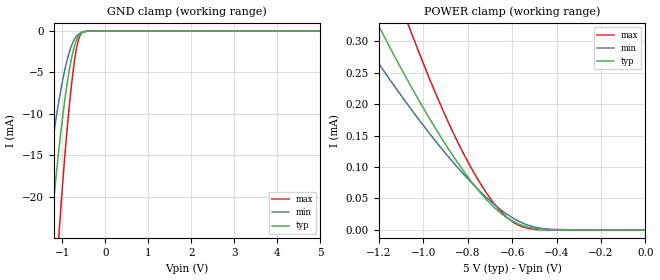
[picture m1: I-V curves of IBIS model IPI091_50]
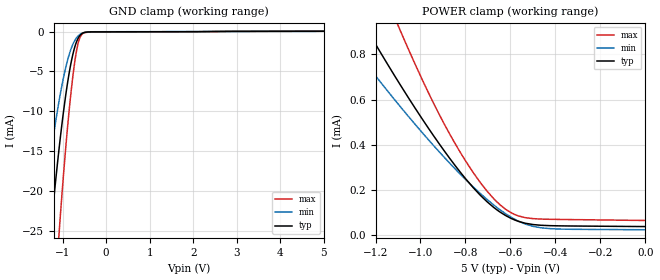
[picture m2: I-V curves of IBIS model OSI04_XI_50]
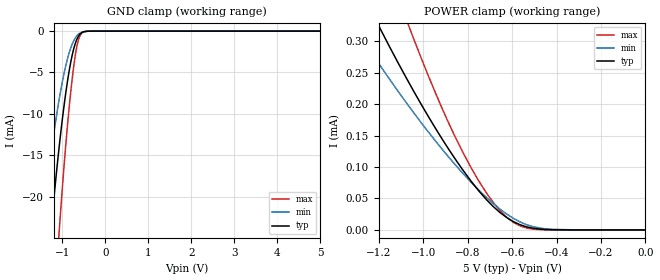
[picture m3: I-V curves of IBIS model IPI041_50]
| TEXAS INSTRUMENTS INCORPORATED
| Connectivity Solutions Group
| IBIS Model of TL16CP752CRHB_5V
| P752C_RHB_5V
| This file contains package information for the following:
|  QFP 32-pin (QFP) package as [Component] P752CRHB_5V
| This device can be powered at the following Vccs:
|  5 Volt Vcc
| This file provides unique models under the [Model Selector] for each Vcc.
| For operation at a specific Vcc, select the appropriate model after each
| [Model Selector] keyword.
[IBIS Ver]   3.2
[Comment char]  |_char
[File Name]   752c_rhb_5v.ibs
[File Rev]   1 | a
[Date]   December 5, 2007
[Source]   Data created from TI-SPICE simulations at TI-CONN.
[Notes]   The following is an IBIS list for the P754C_PM_5V.
   Please contact s-ly@ti.com with questions and
   comments concerning CONN IBIS models.
[Disclaimer] Property of Texas Instruments Incorporated.  Unauthorized
   reproduction and/or distribution is strictly prohibited.
   This product is protected under copyright law.
   Created  2003, (C) Copyright  2003, Texas Instruments
   Incorporated, All Rights Reserved
   UNLESS THERE IS A SIGNED, WRITTEN AGREEMENT TO THE
   CONTRARY, TEXAS INSTRUMENTS (TI) IS PROVIDING THE IBIS
   MODELS  AND WITHOUT ANY WARRANTY, EXPRESSED OR
   IMPLIED.  TI assumes no liability for:
   1) the accuracy of the IBIS models provided to your
   company;
   2) the proper functioning of these IBIS Models in your
   design or for any resulting applications; or
   3) infringement of patents, copyrights or intellectual
   property rights resulting from your use of these IBIS
   models.
   TI provides IBIS Models as a service to our customers.
   You and your company shall not distribute, sell or give
   these models to anyone else without prior written
   permission from TI.
   TI reserves the right to make changes to our products or
   to discontinue any semiconductor product or service
   without notice, and advises our customers to obtain the
   latest version of relevant information to verify, before
   placing orders, that the information being relied on is
   current.
   Please be aware that your receipt and use of the IBIS
   information provided shall serve as acceptance of these
   terms and conditions.  If you do not accept these terms,
   you should return or destroy the IBIS models and any
   other accompanying information immediately.
| Component P754C_5V_QFP 32-pin QFP
[Component]   752C_RHB_5V
[Manufacturer]   Texas Instruments, Inc.
[Package]
|   typ   min   max
R_pkg   0.03169   0.03002   0.03704
L_pkg   2.02289n   1.83543n   2.62435n
C_pkg   0.52087p   0.46196p   0.61212p
[Pin]   signal_name   model_name   R_pin   L_pin   C_pin
1   DSRA   IPI041   0.03729   2.63770n   0.54873p
2   CTSA   IPI041   0.03373   2.35631n   0.61212p
3   DTRA   OPJ430   0.03280   2.22331n   0.58366p
4   VCC   POWER   0.03224   2.13122n   0.55769p
5   RTSA   OPJ430   0.03153   2.03432n   0.53110p
6   INTA   OPJ430   0.03117   1.96768n   0.51149p
7   CSA   IPI041   0.03104   1.92183n   0.49798p
8   TXA   OPJ430   0.03010   1.83593n   0.46505p
9   IOW   IPI041   0.03007   1.83565n   0.46474p
10   TXB   OPJ430   0.03096   1.92107n   0.49718p
11   CSB   IPI041   0.03110   1.96691n   0.51031p
12   INTB   OPJ430   0.03159   2.04484n   0.53228p
13   RTSB   OPJ430   0.03190   2.11324n   0.55339p
14   GND   GND   0.03265   2.22076n   0.58208p
15   DTRB   OPJ430   0.03352   2.34940n   0.60960p
16   CTSB   IPI041   0.03704   2.62435n   0.54475p
17   DSRB   IPI041   0.03652   2.61027n   0.54700p
18   CDB   IPI041   0.03354   2.34759n   0.61094p
19   RIB   IPI041   0.03281   2.22592n   0.58639p
20   RXB   IPI041   0.03222   2.12197n   0.55702p
21   CLKSEL   IPI041   0.03176   2.03735n   0.53446p
22   A2   IPI041   0.03147   1.97163n   0.51867p
23   A1   IPI041   0.03142   1.92513n   0.50753p
24   A0   IPI041   0.03060   1.83543n   0.47574p
25   XTAL1   OSI04_XI   0.03077   1.83703n   0.47632p
26   XTAL2   OSI04   0.03175   1.92839n   0.50935p
27   RESET   IPI091   0.03188   1.96764n   0.51741p
28   GND   GND   0.03231   2.03651n   0.53599p
29   RXC   IPI041   0.03305   2.13263n   0.56045p
30   RIC   IPI041   0.03384   2.23892n   0.58782p
31   CDC   IPI041   0.03485   2.37358n   0.61708p
32   DSRC   IPI041   0.03772   2.62774n   0.54992p
33   CTSC   IPI041   0.03656   2.61266n   0.54247p
34   DTRC   OPJ430   0.03318   2.35035n   0.60872p
35   VCC   POWER   0.03220   2.20948n   0.57926p
36   RTSC   OPJ430   0.03156   2.10738n   0.55066p
37   INTC   OPJ430   0.03109   2.02413n   0.52649p
38   CSC   IPI041   0.03082   1.95908n   0.50691p
39   TXC   OPJ430   0.03074   1.91419n   0.49349p
40   IOR   IPI041   0.03002   1.83657n   0.46196p
41   TXD   OPJ430   0.03011   1.83744n   0.46243p
42   CSD   IPI041   0.03111   1.92648n   0.49841p
43   INTD   OPJ430   0.03138   1.98201n   0.51625p
44   RTSD   OPJ430   0.03165   2.03099n   0.52844p
45   GND   GND   0.03234   2.12591n   0.55667p
46   DTRD   OPJ430   0.03314   2.23103n   0.58547p
47   CTSD   IPI041   0.03404   2.35574n   0.61001p
48   DSRD   IPI041   0.03771   2.63805n   0.54698p
49   CDD   IPI041   0.03740   2.63294n   0.54729p
50   RID   IPI041   0.03400   2.36300n   0.61328p
51   RXD   IPI041   0.03308   2.22978n   0.58494p
52   VCC   POWER   0.03236   2.12568n   0.55651p
53   D0   IPI04_OPJ43   0.03191   2.05000n   0.53623p
54   D1   IPI04_OPJ43   0.03138   1.96454n   0.50911p
55   D2   IPI04_OPJ43   0.03132   1.92758n   0.49950p
56   D3   IPI04_OPJ43   0.03043   1.84011n   0.46416p
57   D4   IPI04_OPJ43   0.03039   1.83956n   0.46402p
58   D5   IPI04_OPJ43   0.03129   1.92740n   0.49881p
59   D6   IPI04_OPJ43   0.03132   1.96376n   0.50826p
60   D7   IPI04_OPJ43   0.03166   2.03022n   0.52764p
61   GND   GND   0.03226   2.12401n   0.55545p
62   RXA   IPI041   0.03290   2.21862n   0.57989p
63   RIA   IPI041   0.03389   2.36071n   0.61163p
64   CDA   IPI041   0.03726   2.62194n   0.54302p
| Model IPI091
[Model Selector]   IPI091
IPI091_50   5 volt Vcc
| Model OSI04_XI
[Model Selector]   OSI04_XI
OSI04_XI_50   5 volt Vcc
| Model IPI041
[Model Selector]   IPI041
IPI041_50   5 volt Vcc
| Model IPI04_OPJ43
[Model Selector]   IPI04_OPJ43
IPI04_OPJ43_50   5 volt Vcc
| Model OPJ430
[Model Selector]   OPJ430
OPJ430_50   5 volt Vcc
| Model OSI04
[Model Selector]   OSI04
OSI04_50   5 volt Vcc
| Models and submodels in the file (6): IPI091_50 (Input), OSI04_XI_50 (Input), IPI041_50 (Input), IPI04_OPJ43_50 (I/O), OPJ430_50 (3-state), OSI04_50 (3-state)
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[Model]   IPI091_50
Model_type  Input
Vinl = 0
Vinh = 5
| variable   typ   min   max
C_comp   1.05pF   0.91pF   1.20pF
[Temperature Range]   40   125   -40
| Ambient temperature   25   110   -40
[Voltage range]   5   4.5   5.5
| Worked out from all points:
|   GND clamp passes 1 mA (typ) near -0.66 V on its own axis
|   POWER clamp passes 1 mA (typ) near -2.02 V on its own axis
[GND Clamp]
| IPI091_50
|   Voltage   I(typ)   I(min)   I(max)
-5V       -337.5mA   -249.9mA   -446.9mA
-1.485V   -37.43mA   -23.94mA   -59.12mA
-1.27V    -24.21mA   -14.96mA   -39.8mA
-1.085V   -14.44mA   -8.531mA   -24.93mA
-1.065V   -13.5mA    -7.923mA   -23.45mA
-920mV    -7.399mA   -4.126mA   -13.63mA
-845mV    -4.864mA   -2.644mA   -9.318mA
-775mV    -2.962mA   -1.595mA   -5.878mA
-665mV    -1.007mA   -578.3uA   -1.875mA
-570mV    -262.1uA   -185.2uA   -368.6uA
-400mV    -8.531uA   -12.92uA   -6.748uA
5V        489.4pA    4.684uA    103.1pA
[POWER Clamp]
| IPI091_50
|   Voltage   I(typ)   I(min)   I(max)
-5V       7.166mA    6.06mA     10.13mA
-1.305V   398.7uA    319.9uA    565.1uA
-1.185V   313.6uA    256.4uA    440.3uA
-1.08V    243.8uA    203.9uA    337.8uA
-1.045V   221.6uA    187.1uA    305.3uA
-915mV    144.4uA    128.2uA    193uA
-785mV    77.58uA    75.9uA     99.02uA
-715mV    47.95uA    51.41uA    58.45uA
-625mV    19.85uA    25.4uA     20.38uA
-565mV    8.395uA    12.83uA    6.553uA
-465mV    1.046uA    2.445uA    370.2nA
-84.4fV   489.4pA    3.799nA    117.2pA
[Model]   OSI04_XI_50
Model_type  Input
Vinl = 0
Vinh = 5
| variable   typ   min   max
C_comp   1.87pF   1.18pF   2.42pF
[Temperature Range]   40   125   -40
| Ambient temperature   25   110   -40
[Voltage range]   5   4.5   5.5
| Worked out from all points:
|   GND clamp passes 1 mA (typ) near -0.66 V on its own axis
|   POWER clamp passes 1 mA (typ) near -1.29 V on its own axis
[GND Clamp]
| OSI04_XI_50
|   Voltage   I(typ)   I(min)   I(max)
-5V       -343.1mA   -253.2mA   -455.7mA
-1.525V   -41.07mA   -26.37mA   -64.46mA
-1.48V    -38.05mA   -24.29mA   -60.12mA
-1.265V   -24.63mA   -15.21mA   -40.45mA
-1.085V   -14.94mA   -8.861mA   -25.7mA
-1.065V   -13.97mA   -8.241mA   -24.18mA
-915mV    -7.534mA   -4.251mA   -13.83mA
-770mV    -3.03mA    -1.696mA   -5.942mA
-665mV    -1.111mA   -697uA     -2.029mA
-565mV    -298uA     -251.7uA   -421.3uA
-390mV    -48.3uA    -40.46uA   -75.23uA
5V        38.17uA    39.29uA    59.24uA
[POWER Clamp]
| OSI04_XI_50
|   Voltage   I(typ)   I(min)   I(max)
-5V       11.35mA    8.695mA    16.41mA
-1.365V   1.132mA    919.8uA    1.585mA
-1.25V    930.2uA    769uA      1.291mA
-1.215V   870.6uA    724.2uA    1.204mA
-1.115V   705.4uA    599.5uA    963.5uA
-1.085V   657.4uA    563.1uA    893.9uA
-945mV    444.6uA    400.2uA    590.1uA
-800mV    250.3uA    246.8uA    329.3uA
-705mV    148.8uA    158.9uA    196uA
-620mV    86.09uA    93.87uA    113.7uA
-465mV    43.98uA    32.94uA    71.4uA
-84.4fV   38.17uA    24.06uA    65.18uA
[Model]   IPI041_50
Model_type  Input
Vinl = 0
Vinh = 5
| variable   typ   min   max
C_comp   1.06pF   0.91pF   1.20pF
[Temperature Range]   40   125   -40
| Ambient temperature   25   110   -40
[Voltage range]   5   4.5   5.5
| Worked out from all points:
|   GND clamp passes 1 mA (typ) near -0.66 V on its own axis
|   POWER clamp passes 1 mA (typ) near -2.02 V on its own axis
[GND Clamp]
| IPI041_50
|   Voltage   I(typ)   I(min)   I(max)
-5V       -337.5mA   -249.9mA   -446.9mA
-1.485V   -37.43mA   -23.94mA   -59.12mA
-1.27V    -24.21mA   -14.96mA   -39.8mA
-1.085V   -14.44mA   -8.531mA   -24.93mA
-1.065V   -13.5mA    -7.923mA   -23.45mA
-920mV    -7.399mA   -4.126mA   -13.63mA
-845mV    -4.864mA   -2.644mA   -9.318mA
-775mV    -2.962mA   -1.595mA   -5.878mA
-665mV    -1.007mA   -578.3uA   -1.875mA
-570mV    -262.1uA   -185.2uA   -368.6uA
-400mV    -8.531uA   -12.92uA   -6.748uA
5V        489.4pA    4.684uA    103.1pA
[POWER Clamp]
| IPI041_50
|   Voltage   I(typ)   I(min)   I(max)
-5V       7.166mA    6.06mA     10.13mA
-1.305V   398.7uA    319.9uA    565.1uA
-1.185V   313.6uA    256.4uA    440.3uA
-1.08V    243.8uA    203.9uA    337.8uA
-1.045V   221.6uA    187.1uA    305.3uA
-915mV    144.4uA    128.2uA    193uA
-785mV    77.58uA    75.9uA     99.02uA
-715mV    47.95uA    51.41uA    58.45uA
-625mV    19.85uA    25.4uA     20.38uA
-565mV    8.395uA    12.83uA    6.553uA
-465mV    1.046uA    2.445uA    370.2nA
-84.4fV   489.4pA    3.799nA    117.2pA
